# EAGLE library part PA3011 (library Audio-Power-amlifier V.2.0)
UNISONIC TECHNOLOGIES As a stereo audio speaker which is operating on a single 5.5V supply, the UTC PA3011 is capable of delivering 3W of output power per channel into 3Ω loads with less than 10% THD+N. The speaker volume level is adjusted by applying a dc voltage to the VOLUME terminal. When a dc voltage is applied, to avoid an unexpected high volume level through the headphones, a third terminal, SEMAX, limits the headphone volume level. And also a fade mode ramps the volume up and down to ensure a smooth transition between active and shutdown modes,. The UTC PA3011 can be applicatated in notebook, LCD monitors and pocket PC.
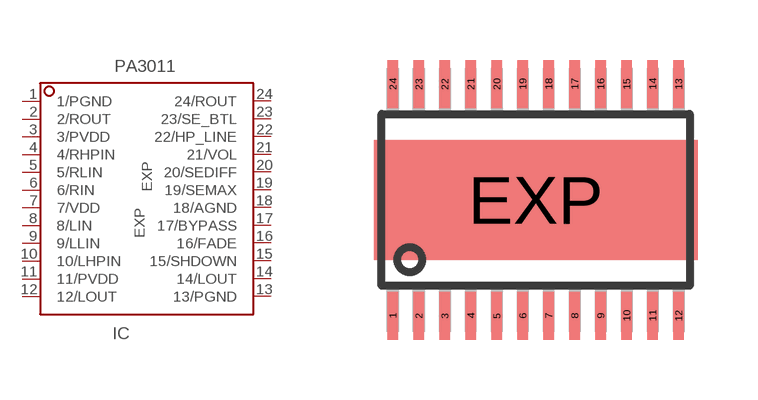
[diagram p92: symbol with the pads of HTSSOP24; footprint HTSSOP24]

Designator prefix IC

## PA3011  [HTSSOP24]
1  1/PGND
2  2/ROUT
3  3/PVDD
4  4/RHPIN
5  5/RLIN
6  6/RIN
7  7/VDD
8  8/LIN
9  9/LLIN
10  10/LHPIN
11  11/PVDD
12  12/LOUT
13  13/PGND
14  14/LOUT
15  15/SHDOWN
16  16/FADE
17  17/BYPASS
18  18/AGND
19  19/SEMAX
20  20/SEDIFF
21  21/VOL
22  22/HP_LINE
23  23/SE_BTL
24  24/ROUT
EXP  EXP

## Footprint HTSSOP24 (pad centres in mm)
HTSSOP24
smd 0.27 x 1.2: 1 -3.575,-2.9; 2 -2.925,-2.9; 3 -2.275,-2.9; 4 -1.625,-2.9; 5 -0.975,-2.9; 6 -0.325,-2.9; 7 0.325,-2.9; 8 0.975,-2.9; 9 1.625,-2.9; 10 2.275,-2.9; 11 2.925,-2.9; 12 3.575,-2.9; 13 3.575,2.9; 14 2.925,2.9; 15 2.275,2.9; 16 1.625,2.9; 17 0.975,2.9; 18 0.325,2.9; 19 -0.325,2.9; 20 -0.975,2.9; 21 -1.625,2.9; 22 -2.275,2.9; 23 -2.925,2.9; 24 -3.575,2.9
smd 8.1 x 3: EXP 0,0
